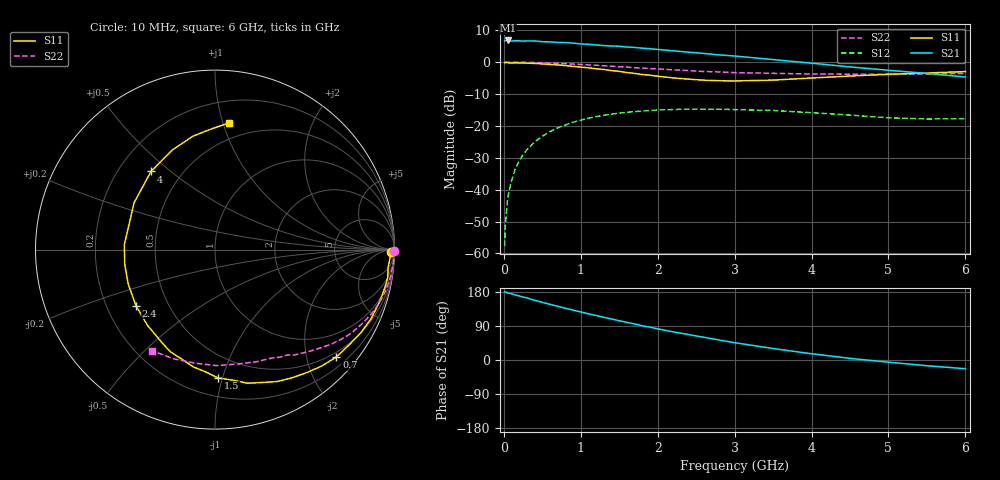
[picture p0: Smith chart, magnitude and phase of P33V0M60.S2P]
! SIEMENS Small Signal Semiconductors
! BFP181
! Si NPN RF Bipolar Junction Transistor in SOT143
! VCE = 3 V  IC = 0.6 mA
! Common Emitter S-Parameters:  March  1996
# GHz  S  MA  R  50
!  f  S11  S21  S12  S22
! GHz  MAG  ANG  MAG  ANG  MAG  ANG  MAG  ANG
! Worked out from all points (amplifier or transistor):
!   36 points, 10 MHz to 6 GHz, reference 50 ohm
!   highest |S21| = 6.8 dB at 50 MHz (marker M1)
!   |S21| within 3 dB of that: start of sweep to 2.086 GHz
!   unconditionally stable (mu >= 1): 3.637 GHz to end of sweep
!   at 250 MHz: K = 0.07, MSG = 17.8 dB, |S12| = -29.0 dB
!   at 1.4 GHz: K = 0.44, MSG = 10.7 dB, |S12| = -16.3 dB
!   at 6 GHz: K = 1.41, MAG = 2.7 dB, |S12| = -17.8 dB
!   S11 on the Smith chart (normalised r, x): 10 MHz: 66, -43; 700 MHz: 0.40, -2.59; 1.5 GHz: 0.33, -0.97; 2.4 GHz: 0.33, -0.29; 4 GHz: 0.34, +0.43; 6 GHz: 0.37, +1.05
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0.01  0.9788 -0.8  2.151 179.7  0.0013 84.3  0.9992 -0.3
0.02  0.9851 -1.2  2.175 179.7  0.0028 82.9  0.9987 -0.5
0.05  0.976 -2.8  2.182 177.3  0.0075 90.5  0.9971 -1.5
0.1  0.9693 -6.0  2.127 174.6  0.0138 84.6  0.9969 -2.9
0.15  0.9747 -9.1  2.157 171.7  0.0214 83.3  0.9961 -4.2
0.25  0.9657 -15.0  2.125 166.1  0.0353 80.3  0.9905 -7.2
0.3  0.961 -18.0  2.149 164.0  0.0423 77.2  0.9903 -8.5
0.4  0.9508 -24.0  2.144 157.6  0.0558 73.6  0.9837 -11.3
0.7  0.9029 -41.5  2.032 141.7  0.0929 61.3  0.9552 -19.4
0.9  0.8562 -53.0  1.985 131.6  0.114 53.3  0.9297 -24.5
1.1  0.8125 -64.8  1.904 121.8  0.1322 46.4  0.9034 -29.1
1.5  0.715 -88.7  1.771 103.6  0.1581 33.8  0.8456 -37.5
1.8  0.6383 -106.7  1.653 90.4  0.1707 25.7  0.8036 -42.9
2.2  0.5652 -131.8  1.503 74.3  0.1803 15.8  0.7559 -49.6
2.4  0.54 -144.7  1.429 67.1  0.1832 11.1  0.7362 -52.9
2.6  0.5203 -158.3  1.365 60.0  0.182 7.6  0.7113 -55.7
3  0.5061 177.0  1.245 45.7  0.18 0.0  0.6832 -62.0
3.5  0.5212 149.8  1.095 30.3  0.1743 -7.1  0.666 -69.8
4  0.5628 129.3  0.962 16.5  0.1609 -12.2  0.6497 -79.0
4.5  0.6039 113.2  0.84 4.4  0.1476 -15.5  0.6463 -89.2
5.5  0.6739 91.4  0.663 -15.1  0.1284 -11.3  0.6503 -110.6
6  0.7104 83.6  0.584 -23.0  0.1292 -7.9  0.6633 -121.7
